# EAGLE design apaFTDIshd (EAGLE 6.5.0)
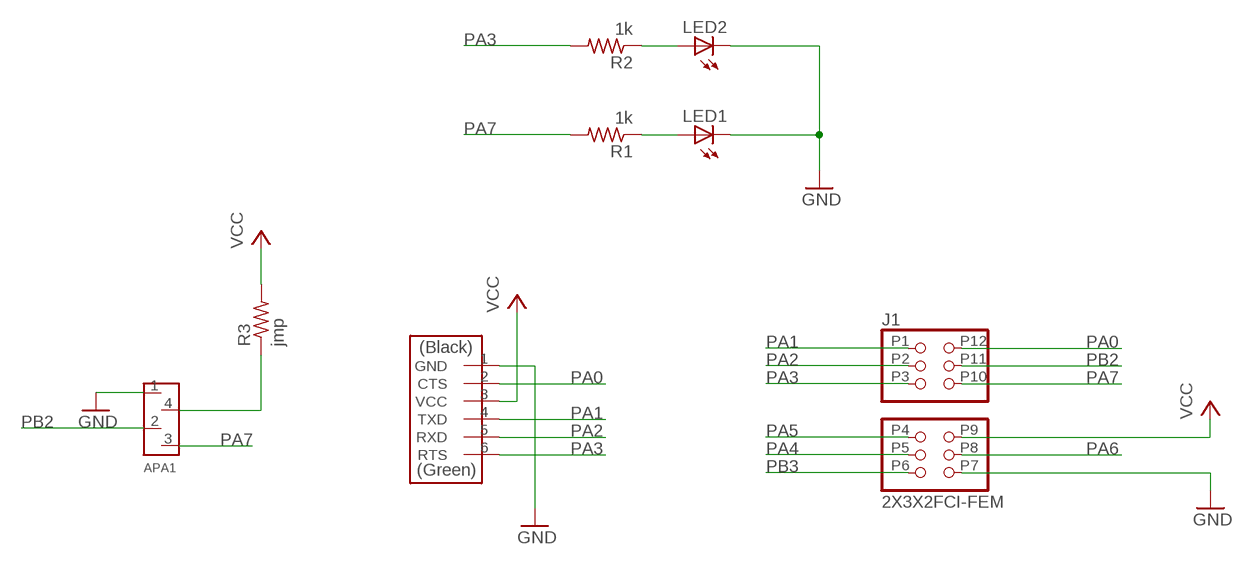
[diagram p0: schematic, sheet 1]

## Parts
APA1  MTA_4MTA_4  [MTA_4]
FTDI  FTDI-SMD-HEADER  [1X06SMD]
J1  2X3X2FCI-FEM  [2X03X2FCI-FEM]
LED1  LED1206  [1206]
LED2  LED1206  [1206]
R1  1k  RESISTOR1206  [1206]
R2  1k  RESISTOR1206  [1206]
R3  jmp  RESISTOR1206  [1206]

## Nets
GND: APA1.1 FTDI.1(GND) J1.P7 LED1.2(C) LED2.2(C)
N$1: LED2.1(A) R2.1
N$2: LED1.1(A) R1.1
N$3: APA1.4 R3.1
PA0: FTDI.2(CTS) J1.P12
PA1: FTDI.4(TXD) J1.P1
PA2: FTDI.5(RXD) J1.P2
PA3: FTDI.6(RTS) J1.P3 R2.2
PA4: J1.P5
PA5: J1.P4
PA6: J1.P8
PA7: APA1.3 J1.P10 R1.2
PB2: APA1.2 J1.P11
PB3: J1.P6
VCC: FTDI.3(VCC) J1.P9 R3.2

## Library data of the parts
APA1 = 01_ng:MTA_4
FTDI = fab:FTDI-SMD-HEADER
J1 = ot:2X3X2FCI-FEM: Use 2 FCI female headers as through hole components on PCB
LED1 LED2 = 01_FAB_Hello:LED
R1-R3 = 01_FAB_Hello:RESISTOR

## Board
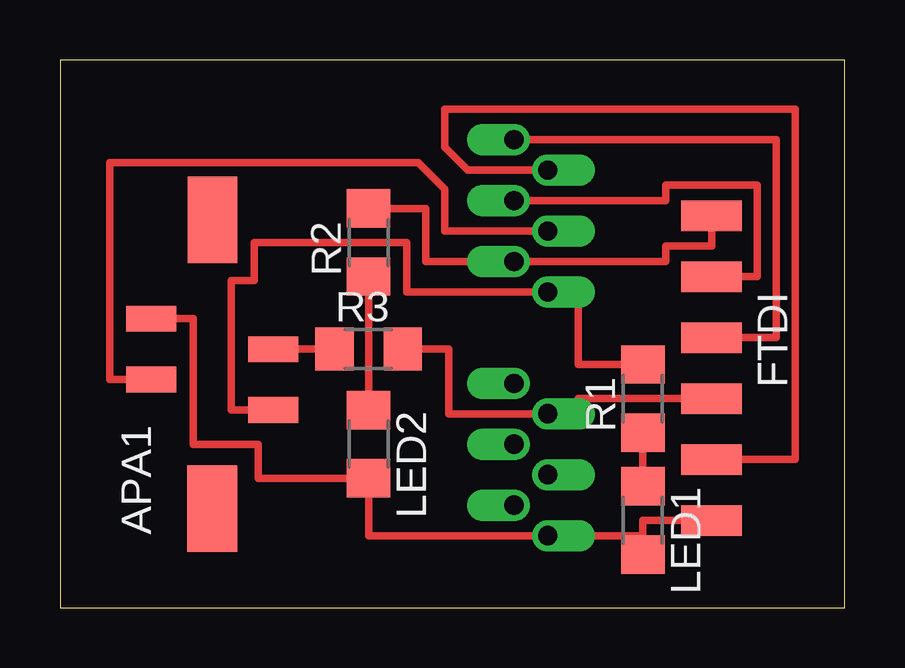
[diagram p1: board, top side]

Size 32.69 x 22.85 mm. Coordinates in mm from the lower left corner, seen from the top.
Outline: 0,0 32.69,0 32.69,22.85 0,22.85 0,0
Copper layers (1*16): Top 0.035mm / dielectric 1.5mm / Bottom 0.035mm
Design rules "default *": minimum track width 10mil, minimum drill 24mil, track to track 0.4mm, track to pad 0.4mm, pad to pad 0.4mm, via to via 0.4mm, smd to smd 0.4mm, copper to edge 40mil, drill to drill 8mil, minimum pad ring 10mil, minimum via ring 8mil, stop-mask expansion 4mil, vias tented up to drill 0mil, thermal gap 10mil

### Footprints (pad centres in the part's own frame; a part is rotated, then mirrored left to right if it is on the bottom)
MTA_4 = smd 1.067 x 2.083: 1 -1.905,-2.54; 2 0.635,-2.54; 3 1.905,2.54; 4 -0.635,2.54 | smd 3.607 x 2.057: P$5 -6.02,0 | smd 3.607 x 2.083: P$6 6.02,0
1X06SMD = smd 2.54 x 1.27: 1 0,6.35; 2 0,3.81; 3 0,1.27; 4 0,-1.27; 5 0,-3.81; 6 0,-6.35
2X03X2FCI-FEM = drill 0.8 pad 1.27 offset: P1 3.045,18.415; P2 3.045,15.875; P3 3.045,13.335; P4 3.045,8.255; P5 3.045,5.715; P6 3.045,3.175; P7 4.445,1.905; P8 4.445,4.445; P9 4.445,6.985; P10 4.445,12.065; P11 4.445,14.605; P12 4.445,17.145
1206 = smd 1.6 x 1.803: 1 -1.422,0; 2 1.422,0

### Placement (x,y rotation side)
APA1  6.35,10.16 270 top
FTDI  27.15,10 180 top
J1  15.88,1.11 0 top
LED1  24.29,3.65 270 top
LED2  12.86,6.83 270 top
R1  24.29,8.73 90 top
R2  12.86,15.24 90 top
R3  12.86,10.79 0 top

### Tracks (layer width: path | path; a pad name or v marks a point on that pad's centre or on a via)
GND
  Top 0.305: APA1.1 5.56,12.06 5.56,6.83 8.26,6.83 8.26,5.4 LED2.2 12.86,3.02 J1.P7 24.29,3.02 | 24.29,3.02 LED1.2 | FTDI.1 24.29,3.65 24.29,3.02
N$1
  Top 0.305: LED2.1 R2.1
N$2
  Top 0.305: LED1.1 R1.1
N$3
  Top 0.305: APA1.4 R3.1
PA0
  Top 0.305: J1.P12 16.99,18.26 16.03,19.21 16.03,20.8 30.64,20.8 30.64,6.19 FTDI.2
PA1
  Top 0.305: J1.P1 29.84,19.53 29.84,11.27 FTDI.4
PA2
  Top 0.305: J1.P2 25.24,16.99 25.24,17.62 29.05,17.62 29.05,13.81 FTDI.5
PA3
  Top 0.305: R2.2 15.24,16.66 15.24,14.45 J1.P3 25.24,14.45 25.24,15.08 27.15,15.08 FTDI.6
PA7
  Top 0.305: APA1.3 7.14,8.26 7.14,13.65 8.1,13.65 8.1,15.24 14.45,15.24 14.45,13.18 J1.P10 21.59,13.18 21.59,10.15 R1.2
PB2
  Top 0.305: APA1.2 2.06,9.53 2.06,18.57 14.92,18.57 16.03,17.46 16.03,15.72 J1.P11
VCC
  Top 0.305: R3.2 16.19,10.79 16.19,8.1 J1.P9 21.59,8.1 21.59,8.73 FTDI.3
